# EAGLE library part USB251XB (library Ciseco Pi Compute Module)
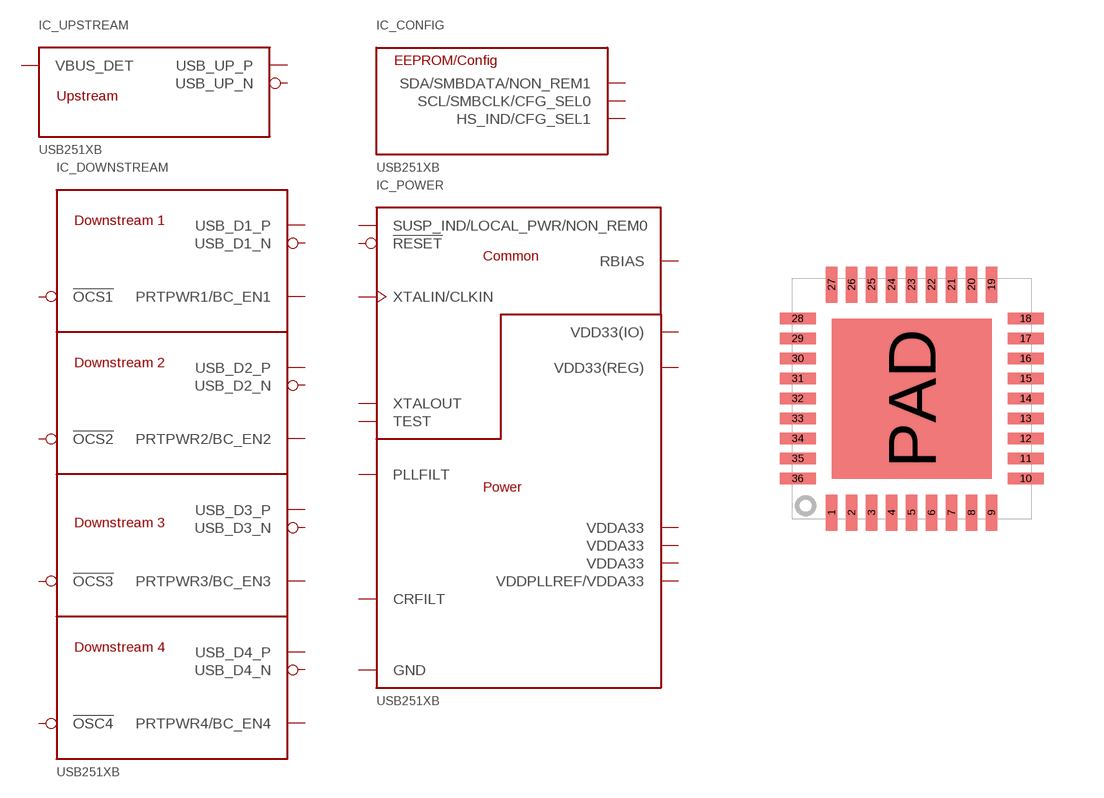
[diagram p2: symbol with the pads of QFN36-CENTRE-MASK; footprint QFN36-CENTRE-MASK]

Designator prefix IC; gates _UPSTREAM=USB251XB_UPSTREAM _DOWNSTREAM=USB251XB_DOWNSTREAM _CONFIG=USB251XB_EEPROM _POWER=USB251XB_POWER

## USB251XB  [QFN36-CENTRE-MASK]
1  _DOWNSTREAM:USB_D1_N
2  _DOWNSTREAM:USB_D1_P
3  _DOWNSTREAM:USB_D2_N
4  _DOWNSTREAM:USB_D2_P
5  _POWER:VDDA33  pwr
6  _DOWNSTREAM:USB_D3_N
7  _DOWNSTREAM:USB_D3_P
8  _DOWNSTREAM:USB_D4_N
9  _DOWNSTREAM:USB_D4_P
10  _POWER:VDDA33  pwr
11  _POWER:TEST
12  _DOWNSTREAM:PRTPWR1/BC_EN1
13  _DOWNSTREAM:!OCS1  in
14  _POWER:CRFILT
15  _POWER:VDD33(REG)  pwr
16  _DOWNSTREAM:PRTPWR2/BC_EN2
17  _DOWNSTREAM:!OCS2  in
18  _DOWNSTREAM:PRTPWR3/BC_EN3
19  _DOWNSTREAM:!OCS3  in
20  _DOWNSTREAM:PRTPWR4/BC_EN4
21  _DOWNSTREAM:!OSC4  in
22  _CONFIG:SDA/SMBDATA/NON_REM1
23  _POWER:VDD33(IO)  pwr
24  _CONFIG:SCL/SMBCLK/CFG_SEL0
25  _CONFIG:HS_IND/CFG_SEL1
26  _POWER:!RESET
27  _UPSTREAM:VBUS_DET
28  _POWER:SUSP_IND/LOCAL_PWR/NON_REM0
29  _POWER:VDDA33  pwr
30  _UPSTREAM:USB_UP_N
31  _UPSTREAM:USB_UP_P
32  _POWER:XTALOUT
33  _POWER:XTALIN/CLKIN
34  _POWER:PLLFILT
35  _POWER:RBIAS
36  _POWER:VDDPLLREF/VDDA33  pwr
PAD  _POWER:GND  pwr

## Footprint QFN36-CENTRE-MASK (pad centres in mm)
smd 0.28 x 0.9: 1 -2,-2.85; 2 -1.5,-2.85; 3 -1,-2.85; 4 -0.5,-2.85; 5 0,-2.85; 6 0.5,-2.85; 7 1,-2.85; 8 1.5,-2.85; 9 2,-2.85; 19 2,2.85; 20 1.5,2.85; 21 1,2.85; 22 0.5,2.85; 23 0,2.85; 24 -0.5,2.85; 25 -1,2.85; 26 -1.5,2.85; 27 -2,2.85
smd 0.9 x 0.28: 10 2.85,-2; 11 2.85,-1.5; 12 2.85,-1; 13 2.85,-0.5; 14 2.85,0; 15 2.85,0.5; 16 2.85,1; 17 2.85,1.5; 18 2.85,2; 28 -2.85,2; 29 -2.85,1.5; 30 -2.85,1; 31 -2.85,0.5; 32 -2.85,0; 33 -2.85,-0.5; 34 -2.85,-1; 35 -2.85,-1.5; 36 -2.85,-2
smd 4 x 4: PAD 0,0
